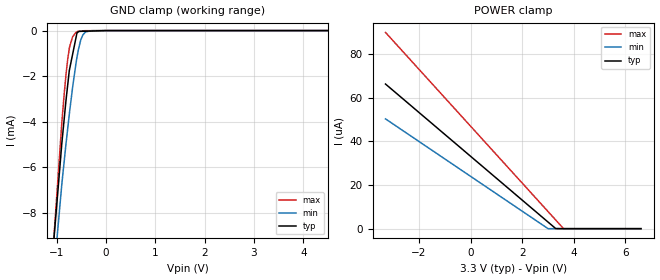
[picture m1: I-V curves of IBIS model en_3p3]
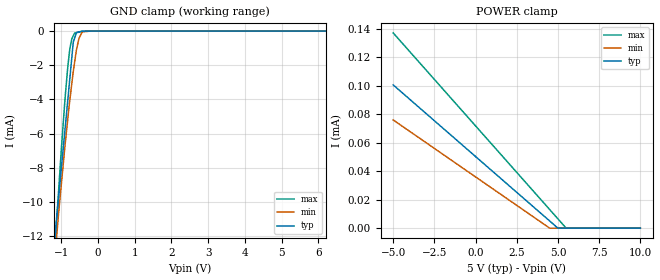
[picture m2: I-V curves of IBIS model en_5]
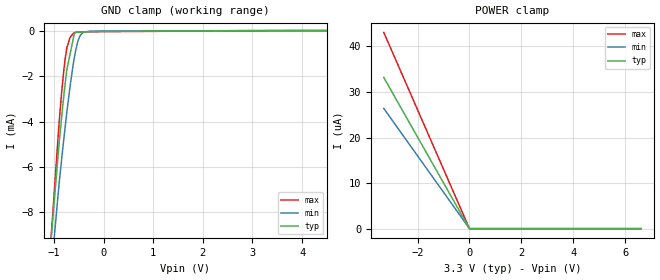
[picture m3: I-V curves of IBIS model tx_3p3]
|Texas Instruments Incorporated
| IO-LINK PHY for Device Nodes
| Marketing part#   Digital Voltage Range   Package-type   #pins
| SN65HVD101   3.0V-5.5V   PVQFN   20
[IBIS Ver]   4.1
[File name]   sn65hvd101.ibs
[File Rev]   1.0
[Date]   2/18/2013
[Source]
| Texas Instruments Incorporated.
| Analog-eLab Design Center, HPA
| 12500 TI Blvd
| Dallas, TX -75243
[Notes]   Revision History:
| Rev 1.0: 2/18/2013
| - Initial version of the model
| - Model generated from simulations in TISPICE
| - Model matched to SPICE simulation
| - C_comp although listed in numerical order of value are
|   obtained from varying PVT conditions. For PVT conditions for
|   each specific value refer the buffer description under
|   respective [Model]. IBIS model user is responsible for using
|   appropriate C_comp to simulate for Signal Integrity.
| - Model names with a trailing _3p3 contains the model for
|   3.3V [3V and 3.6V].Model names with a trailing _5 contains
|   the model for 5V [4.5V and 5.5V].
|*  EXCEPTION:   *
|*  - For model en_*, there will be leakage current in the POWER clamp  *
|*   I-V Table because of pulldown resistor (R1) connected on pad.   *
|*  - For model tx_*, there will be leakage current in the GND clamp   *
|*   I-V Table because of the pullup resistor (R2) connected on pad.   *
|*  - For model vcc_*, there will be leakage current in the GND clamp   *
|*   I-V Table because of the pullup resistor (R0) connected on pad.   *
[Disclaimer]
| This model is designed as an aid for customers of Texas Instruments.
| TI and its licensors and suppliers make no warranties, either expressed
| or implied, with respect to this  model, including the warranties of
| merchantability or fitness for a particular purpose. The model is
| provided solely on an "as is" basis. The entire risk as to its quality
| and performance is with the customer.
[Copyright]
(C) Copyright 2013 Texas Instruments Incorporated.All rights reserved.
|   SN65HVD101RGB
[Component]   SN65HVD101RGB
[Manufacturer]   TI
[Package]   |20 PVQFN  -  RGB package
|   typ   min   max
R_pkg   0.05612   0.05272   0.06249
L_pkg   0.93421nH   0.87397nH   1.05588nH
C_pkg   0.12936pF   0.12096pF   0.13785pF
[Pin]  signal_name   model_name   R_pin   L_pin   C_pin
1   Vcc_SET   VCC   0.05379   0.89355nH  0.12222pF
2   NC   NC   0.00018   0.03410nH  0.08028pF
3   GND   GND   0.02644   0.57753nH  0.16089pF
4   ILIM_ADJ   NC   0.05905   0.99187nH  0.14222pF
5   PWR_OK   PWR_CUR   0.05272   0.87397nH  0.12096pF
6   GND   GND   0.05900   0.98896nH  0.12871pF
7   Vcc_IN   POWER   0.05703   0.95045nH  0.14020pF
8   Vcc_OUT   NC   0.05964   0.99804nH  0.14319pF
9   NC   NC   0.00018   0.03410nH  0.08028pF
10   L+   POWER   0.03670   0.94311nH  0.16772pF
11   NC   NC   0.00018   0.03468nH  0.06688pF
12   CQ   NC   0.02913   0.66827nH  0.16980pF
13   GND   GND   0.05675   0.94109nH  0.14425pF
14   L-   GND   0.06635   1.12650nH  0.15275pF
15   CUR_OK   PWR_CUR   0.05577   0.92370nH  0.12223pF
16   WAKE   WAKE   0.05823   0.97137nH  0.12608pF
17   RX   RX   0.05499   0.91088nH  0.13685pF
18   TX   TX   0.05440   0.90109nH  0.13622pF
19   TEMP_OK   OK   0.05658   0.94327nH  0.13785pF
20   EN   EN   0.06249   1.05588nH  0.13247pF
|   Model Selectors
[Model Selector] EN
en_3p3   3.3V  digital input
en_5   5.0V  digital input
[Model Selector] TX
tx_3p3  3.3V  digital input
tx_5   5.0V  digital input
[Model Selector] VCC
vcc_3p3   3.3V  digital input
vcc_5   5.0V  digital input
[Model Selector] RX
rx_3p3   3.3V  digital output
rx_5   5.0V  digital output
[Model Selector] OK
ok_3p3   3.3V  digital open_drain
ok_5   5.0V  digital open_drain
[Model Selector] PWR_CUR
pwr_cur_3p3   3.3V  digital open_drain
pwr_cur_5   5.0V  digital open_drain
[Model Selector] WAKE
wake_3p3   3.3V  digital open_drain
wake_5   5.0V  digital open_drain
| Models and submodels in the file (14): en_3p3 (Input), en_5 (Input), tx_3p3 (Input), tx_5 (Input), vcc_3p3 (Input), vcc_5 (Input), rx_3p3 (Output), rx_5 (Output), ok_3p3 (Open_drain), ok_5 (Open_drain), pwr_cur_3p3 (Open_drain), pwr_cur_5 (Open_drain), wake_3p3 (Open_drain), wake_5 (Open_drain)
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|   en_3p3 Model
[Model]   en_3p3
Model_type   Input
Vinl = 0.8
Vinh = 2.0
|   typ   min   max
|   (nom PVT)   (fast PVT)   (slow PVT)
C_comp   8.028e-13   7.642e-13   8.321e-13
| Where nom  PVT is Nominal Process, 3.3V, 45C
|   Fast PVT is Strong Process,  3.6V, -20C
|   Slow PVT is Weak Process,   3V, 125C
[Voltage Range]   3.3   3   3.6
|Junction Temperature
[Temperature Range]   45   125   -20
[Power Clamp Reference]   3.3   3   3.6
[GND Clamp Reference]   0   0   0
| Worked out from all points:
|   GND clamp passes 1 mA (typ) near -0.67 V on its own axis
[GND Clamp]
|   Voltage   I(typ)   I(min)   I(max)
-3.3V     -95.27mA   -81.25mA   -114.6mA
-1.127V   -10.95mA   -12.3mA    -11.22mA
-897.6mV  -4.956mA   -6.741mA   -4.043mA
-849.6mV  -3.881mA   -5.736mA   -2.785mA
-777.6mV  -2.375mA   -4.289mA   -1.251mA
-745.8mV  -1.754mA   -3.676mA   -786.6uA
-676.8mV  -1.022mA   -2.462mA   -262.1uA
-590.7mV  -108.3uA   -1.184mA   -56.74uA
-572.4mV  -72.55uA   -968.6uA   -36.08uA
-471mV    -30.87uA   -188.5uA   -13.4uA
-285mV    -18.61uA   -4.121uA   -3.844uA
6.6V      0A         0A         0A
[POWER Clamp]
|   Voltage   I(typ)   I(min)   I(max)
-3.3V     66.37uA    50.38uA    90.06uA
2.997V    3.047uA    24.03nA    7.871uA
3.297V    33.18nA    0A         3.959uA
3.596V    0A         0A         46.99nA
6.6V      0A         0A         0A
|   en_5 Model
[Model]   en_5
Model_type   Input
Vinl = 0.8
Vinh = 2.0
|   typ   min   max
|   (nom PVT)   (fast PVT)   (slow PVT)
C_comp   8.085e-13   7.971e-13   8.143e-13
| Where nom  PVT is Nominal Process, 5V, 45C
|   Fast PVT is Strong Process,  5.5V, -20C
|   Slow PVT is Weak Process,   4.5V, 125C
[Voltage Range]   5   4.5   5.5
|Junction Temperature
[Temperature Range]   45   125   -20
[Power Clamp Reference]   5   4.5   5.5
[GND Clamp Reference]   0   0   0
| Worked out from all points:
|   GND clamp passes 1 mA (typ) near -0.69 V on its own axis
[GND Clamp]
|   Voltage   I(typ)   I(min)   I(max)
-5V       -180.5mA   -153.1mA   -213.9mA
-1.14V    -11.31mA   -12.44mA   -11.7mA
-1.105V   -10.53mA   -11.57mA   -10.5mA
-907.5mV  -6.03mA    -6.954mA   -4.312mA
-819.5mV  -4.03mA    -5.126mA   -2.08mA
-759mV    -2.656mA   -3.94mA    -959.1uA
-670mV    -634uA     -2.347mA   -272.1uA
-632.5mV  -395.5uA   -1.798mA   -120.2uA
-517.5mV  -49.09uA   -440.8uA   -64.34uA
-441mV    -8.568uA   -101.9uA   -27.16uA
-202.5mV  -2.509uA   -1.796uA   -2.704uA
10V       0A         0A         0A
[POWER Clamp]
|   Voltage   I(typ)   I(min)   I(max)
-5V       100.6uA    75.97uA    137uA
4.495V    5.073uA    36.05nA    13.11uA
4.995V    50.28nA    0A         6.591uA
5.495V    0A         0A         71.79nA
10V       0A         0A         0A
|   tx_3p3 Model
[Model]   tx_3p3
Model_type   Input
Vinl = 0.8
Vinh = 2.0
|   typ   min   max
|   (nom PVT)   (fast PVT)   (slow PVT)
C_comp   8.028e-13   7.642e-13   8.321e-13
| Where nom  PVT is Nominal Process, 3.3V, 45C
|   Fast PVT is Strong Process,  3.6V, -20C
|   Slow PVT is Weak Process,   3V, 125C
[Voltage Range]   3.3   3   3.6
|Junction Temperature
[Temperature Range]   45   125   -20
[Power Clamp Reference]   3.3   3   3.6
[GND Clamp Reference]   0   0   0
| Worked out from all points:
|   GND clamp passes 1 mA (typ) near -0.67 V on its own axis
[GND Clamp]
|   Voltage   I(typ)   I(min)   I(max)
-3.3V     -95.3mA    -81.27mA   -114.7mA
-1.127V   -10.98mA   -12.32mA   -11.27mA
-897.6mV  -4.99mA    -6.765mA   -4.09mA
-849.6mV  -3.914mA   -5.76mA    -2.832mA
-777.6mV  -2.409mA   -4.313mA   -1.298mA
-745.8mV  -1.788mA   -3.7mA     -833.6uA
-676.8mV  -1.055mA   -2.486mA   -309.1uA
-590.7mV  -141.5uA   -1.208mA   -103.7uA
-572.4mV  -105.7uA   -992.6uA   -83.07uA
-471mV    -64.06uA   -212.5uA   -60.39uA
-285mV    -51.79uA   -28.11uA   -50.83uA
6.6V      0A         0A         0A
[POWER Clamp]
|   Voltage   I(typ)   I(min)   I(max)
-3.3V     33.19uA    26.39uA    43.07uA
-59.4mV   597.4nA    475.7nA    775.4nA
-33.83fV  0A         0A         0A
6.6V      0A         0A         0A
